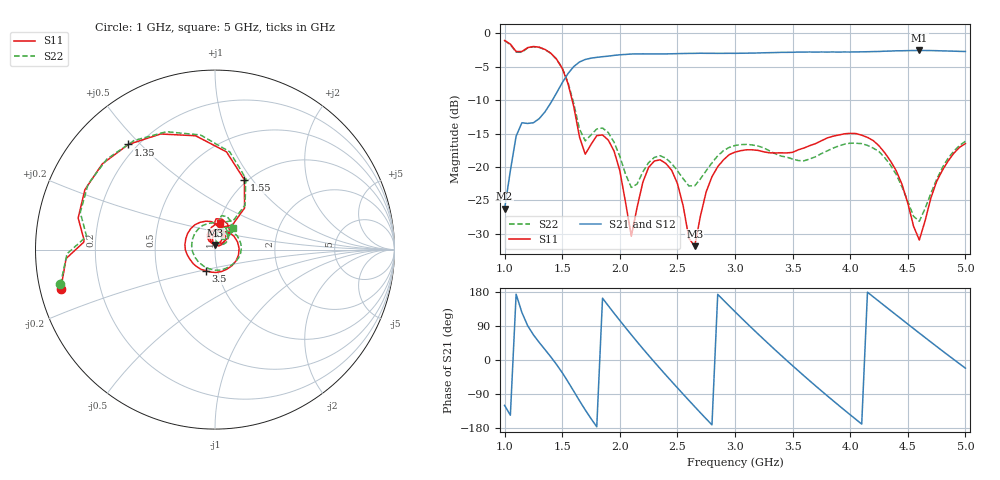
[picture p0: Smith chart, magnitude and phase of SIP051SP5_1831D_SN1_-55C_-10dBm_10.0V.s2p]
# GHz  S  dB  R  50
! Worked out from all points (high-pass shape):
!   81 points, 1 GHz to 5 GHz, reference 50 ohm
!   highest |S21| = -2.55 dB at 4.6 GHz (marker M1); lowest = -26.3 dB at 1 GHz (marker M2)
!   |S21| within 3 dB of the highest: 1.572 GHz to end of sweep
!   lowest |S11| = -31.9 dB at 2.65 GHz (marker M3), VSWR 1.05, Z = 50.1 + j2.56 ohm
!   |S11| at or under -10 dB: 1.587 GHz to end of sweep
!   |S22| runs from -28.1 to -1.1 dB; largest |S21 - S12| = 0.0021
!   S11 on the Smith chart (normalised r, x): 1 GHz: 0.06, -0.12; 1.35 GHz: 0.17, +0.46; 1.55 GHz: 0.97, +0.91; 3.5 GHz: 0.88, -0.21; 5 GHz: 1.01, +0.30
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1  -1.05 -165.8  -26.26 -119.8  -26.26 -119.4  -1.08 -167.3
1.1  -2.71 176.7  -15.38 173.6  -15.36 173.6  -2.81 174.5
1.35  -2.40 129.5  -11.76 27.7  -11.75 27.6  -2.42 126.7
1.55  -7.49 67.2  -6.02 -57.2  -6.02 -57.2  -7.31 66.5
1.7  -18.09 77.6  -3.90 -131.7  -3.90 -131.8  -16.08 74.4
1.85  -15.20 76.9  -3.48 163.1  -3.48 163.1  -14.16 70.3
2.05  -25.32 42.3  -3.15 85.3  -3.15 85.3  -21.08 46.1
2.1  -30.34 80.0  -3.08 66.6  -3.09 66.6  -23.06 60.6
2.35  -18.92 79.4  -3.06 -22.7  -3.07 -22.6  -18.30 64.6
2.5  -22.46 42.3  -3.03 -73.5  -3.02 -73.5  -20.54 45.0
2.65  -31.85 86.6  -2.99 -123.0  -2.99 -123.0  -22.82 60.3
2.8  -21.46 93.4  -2.98 -171.1  -2.97 -171.1  -19.38 63.7
3  -17.77 34.7  -2.98 127.4  -2.97 127.5  -16.77 32.4
3.2  -17.51 -28.3  -2.93 68.7  -2.92 68.8  -16.84 -9.0
3.5  -17.80 -113.5  -2.82 -15.1  -2.82 -15.1  -18.80 -90.2
3.7  -16.49 -158.6  -2.80 -68.4  -2.79 -68.4  -18.45 -158.6
3.85  -15.39 170.6  -2.78 -106.9  -2.78 -107.0  -17.19 155.9
4.05  -14.99 129.1  -2.77 -156.8  -2.77 -156.9  -16.44 104.2
4.35  -19.10 69.0  -2.64 130.7  -2.65 130.7  -19.71 43.1
4.6  -30.93 92.9  -2.55 71.1  -2.56 71.1  -28.12 65.7
4.8  -20.50 116.7  -2.62 24.2  -2.61 24.2  -20.10 81.5
5  -16.50 79.6  -2.70 -21.6  -2.72 -21.6  -16.14 49.5
